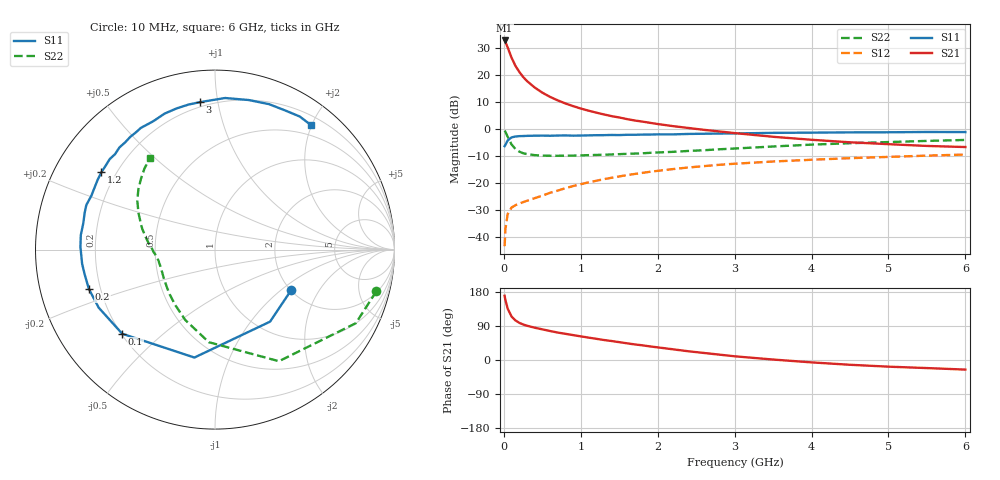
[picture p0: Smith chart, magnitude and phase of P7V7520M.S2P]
! SIEMENS Small Signal Semiconductors
! BFP196
! Si NPN RF Bipolar Junction Transistor in SOT143
! VCE = 0.75 V  IC = 20 mA
! Common Emitter S-Parameters:  May  1996
# GHz  S  MA  R  50
!  f  S11  S21  S12  S22
! GHz  MAG  ANG  MAG  ANG  MAG  ANG  MAG  ANG
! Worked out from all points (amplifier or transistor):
!   36 points, 10 MHz to 6 GHz, reference 50 ohm
!   highest |S21| = 32.8 dB at 10 MHz (marker M1)
!   |S21| within 3 dB of that: start of sweep to 55.38 MHz
!   unconditionally stable (mu >= 1): 597.1 MHz to end of sweep
!   at 250 MHz: K = 0.62, MSG = 23.2 dB, |S12| = -27.2 dB
!   at 1.4 GHz: K = 1.12, MAG = 9.3 dB, |S12| = -18.1 dB
!   at 6 GHz: K = 1.02, MAG = 0.5 dB, |S12| = -9.5 dB
!   S11 on the Smith chart (normalised r, x): 10 MHz: 2.00, -1.18; 100 MHz: 0.20, -0.37; 200 MHz: 0.16, -0.15; 1.2 GHz: 0.15, +0.30; 3 GHz: 0.17, +0.89; 6 GHz: 0.34, +2.00
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0.01  0.4807 -28.2  43.79 169.6  0.0067 81.0  0.9286 -14.5
0.02  0.5052 -52.6  41.14 158.6  0.0138 69.5  0.8853 -27.6
0.05  0.6122 -100.8  32.49 135.5  0.0264 52.3  0.7167 -60.2
0.1  0.6979 -137.8  21.01 114.9  0.0348 39.2  0.5171 -93.8
0.15  0.7243 -153.5  14.88 104.6  0.0385 35.8  0.4257 -112.9
0.2  0.736 -162.6  11.5 98.2  0.0412 36.0  0.3801 -125.7
0.25  0.7392 -169.2  9.238 93.8  0.0439 37.1  0.3552 -135.2
0.3  0.7446 -173.9  7.757 90.5  0.0465 38.9  0.3418 -141.3
0.4  0.7499 178.9  5.884 85.3  0.052 42.6  0.3271 -150.5
0.5  0.7521 173.8  4.717 80.9  0.058 45.3  0.3205 -156.6
0.6  0.7483 168.9  3.942 76.5  0.0653 48.0  0.3183 -160.6
0.7  0.7548 164.0  3.391 72.4  0.0719 48.8  0.3181 -163.7
0.9  0.7514 156.5  2.653 65.7  0.0872 50.3  0.32 -168.5
1.1  0.7607 149.3  2.185 59.1  0.1023 50.5  0.3269 -171.9
1.2  0.7658 145.7  2.01 56.0  0.1093 50.1  0.3296 -173.5
1.7  0.7797 129.8  1.437 41.1  0.1462 46.0  0.3493 179.6
2.2  0.7935 115.8  1.128 28.2  0.1804 40.1  0.3765 173.3
3  0.8256 95.9  0.838 9.8  0.2265 29.4  0.4336 161.6
3.5  0.8465 86.2  0.716 1.2  0.2491 23.0  0.4728 154.4
4.5  0.8645 69.6  0.566 -12.6  0.2871 11.5  0.5437 141.7
5.5  0.8791 57.5  0.484 -21.3  0.3201 0.8  0.6005 130.7
6  0.8759 52.2  0.462 -25.3  0.335 -5.0  0.6255 125.1
